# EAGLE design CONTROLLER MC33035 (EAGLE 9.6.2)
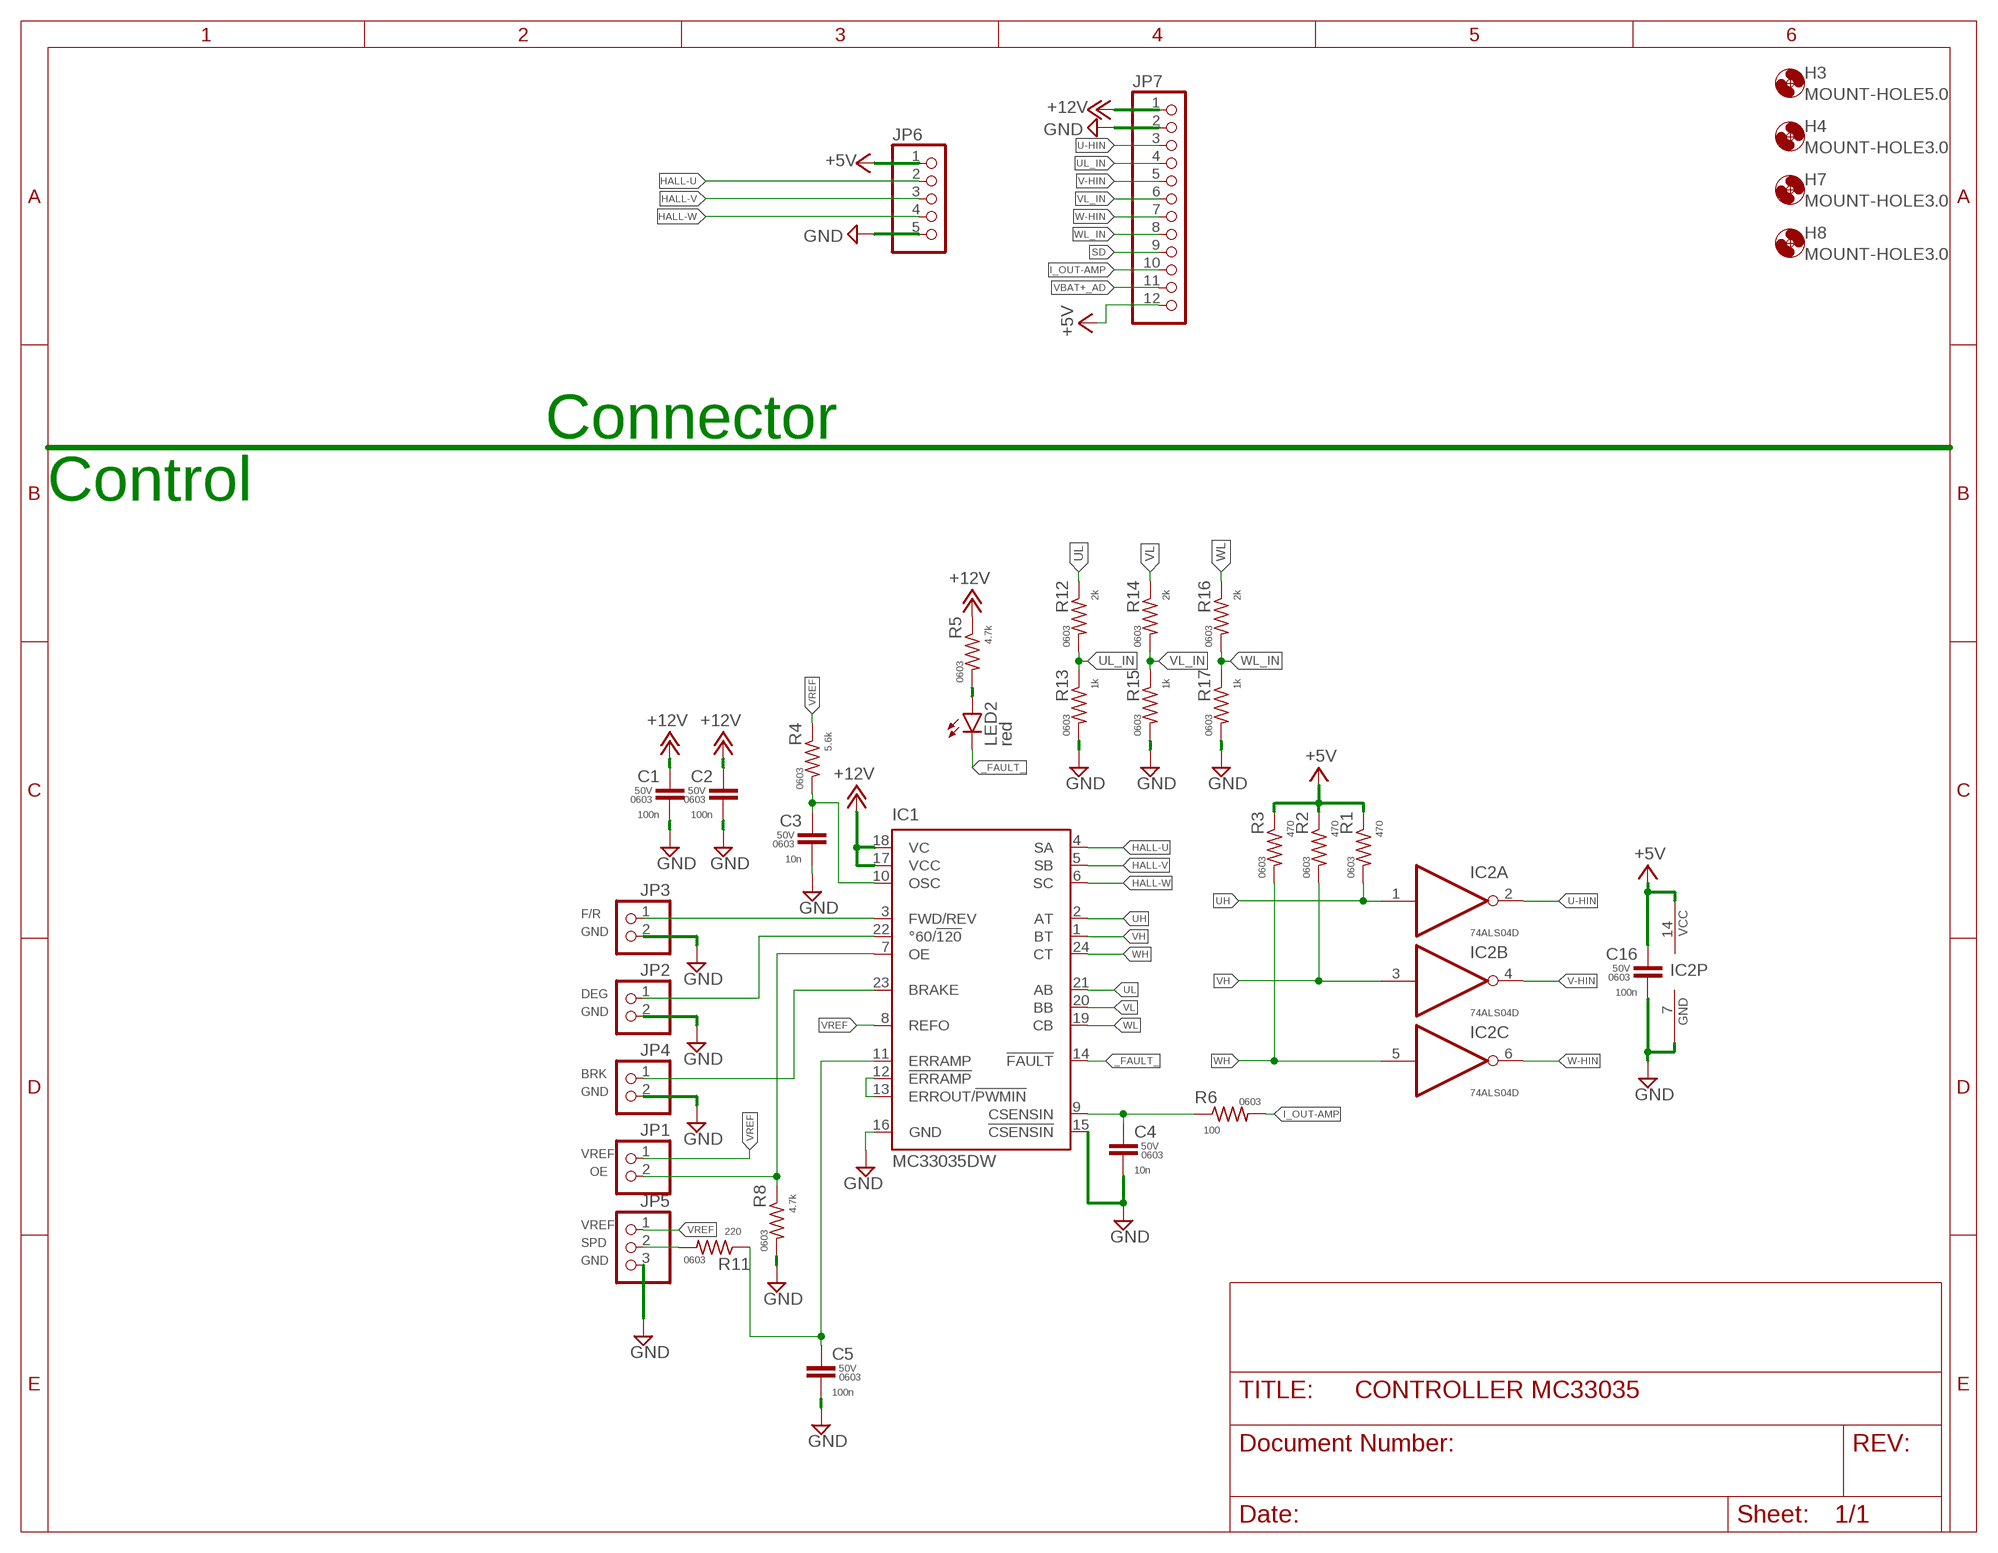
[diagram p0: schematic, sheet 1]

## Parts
C1  100n  C-EUC0603  [C0603]
C2  100n  C-EUC0603  [C0603]
C3  10n  C-EUC0603  [C0603]
C4  10n  C-EUC0603  [C0603]
C5  100n  C-EUC0603  [C0603]
C16  100n  C-EUC0603  [C0603]
H3  MOUNT-HOLE5.0  [5,0]
H4  MOUNT-HOLE3.0  [3,0]
H7  MOUNT-HOLE3.0  [3,0]
H8  MOUNT-HOLE3.0  [3,0]
IC1  MC33035DW  [SO24L]
IC2  74ALS04D  [SO14]
JP1  PINHD-1X2  [1X02]
JP2  PINHD-1X2  [1X02]
JP3  PINHD-1X2  [1X02]
JP4  PINHD-1X2  [1X02]
JP5  PINHD-1X3  [1X03]
JP6  PINHD-1X5  [1X05]
JP7  PINHD-1X12  [1X12]
LED2  red  LEDCHIP-LED0805  [CHIP-LED0805]
R1  470  R-US_R0603  [R0603]
R2  470  R-US_R0603  [R0603]
R3  470  R-US_R0603  [R0603]
R4  5.6k  R-US_R0603  [R0603]
R5  4.7k  R-US_R0603  [R0603]
R6  100  R-US_R0603  [R0603]
R8  4.7k  R-US_R0603  [R0603]
R11  220  R-US_R0603  [R0603]
R12  2k  R-US_R0603  [R0603]
R13  1k  R-US_R0603  [R0603]
R14  2k  R-US_R0603  [R0603]
R15  1k  R-US_R0603  [R0603]
R16  2k  R-US_R0603  [R0603]
R17  1k  R-US_R0603  [R0603]

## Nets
+5V: C16.1 IC2.14(P:VCC) JP6.1 JP7.12 R1.1 R2.1 R3.1
+12V: C1.1 C2.1 IC1.17(VCC) IC1.18(VC) JP7.1 R5.1
_FAULT_: IC1.14(!FAULT) LED2.C
BRK: IC1.23(BRAKE) JP4.1
CSENSE: C4.1 IC1.9(CSENSIN) R6.1
DEG: IC1.22(°60/!120) JP2.1
F/R: IC1.3(FWD/REV) JP3.1
GND: C1.2 C2.2 C3.2 C4.2 C5.2 C16.2 IC1.15(!CSENSIN) IC1.16(GND) IC2.7(P:GND) JP2.2 JP3.2 JP4.2 JP5.3 JP6.5 JP7.2 R8.2 R13.2 R15.2 R17.2
HALL-U: IC1.4(SA) JP6.2
HALL-V: IC1.5(SB) JP6.3
HALL-W: IC1.6(SC) JP6.4
I_OUT-AMP: JP7.10 R6.2
N$2: LED2.A R5.2
N$3: JP5.2 R11.2
N$6: IC1.12(!ERRAMP) IC1.13(ERROUT/!PWMIN)
OE: IC1.7(OE) JP1.2 R8.1
OSC: C3.1 IC1.10(OSC) R4.2
SD: JP7.9
SPD: C5.1 IC1.11(ERRAMP) R11.1
U-HIN: IC2.2(A:O) JP7.3
UH: IC1.2(AT) IC2.1(A:I) R1.2
UL: IC1.21(AB) R12.1
UL_IN: JP7.4 R12.2 R13.1
V-HIN: IC2.4(B:O) JP7.5
VBAT+_AD: JP7.11
VH: IC1.1(BT) IC2.3(B:I) R2.2
VL: IC1.20(BB) R14.1
VL_IN: JP7.6 R14.2 R15.1
VREF: IC1.8(REFO) JP1.1 JP5.1 R4.1
W-HIN: IC2.6(C:O) JP7.7
WH: IC1.24(CT) IC2.5(C:I) R3.2
WL: IC1.19(CB) R16.1
WL_IN: JP7.8 R16.2 R17.1
Unconnected: IC2.8(D:O) IC2.9(D:I) IC2.10(E:O) IC2.11(E:I) IC2.12(F:O) IC2.13(F:I)

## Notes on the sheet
- Connector
- Control

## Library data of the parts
C1-C5 C16 = rcl:C-EU: CAPACITOR, European symbol; SIZE: 0603; SPICEPREFIX: C; VOLTAGE: 50V
H3 H4 H7 H8 = holes:MOUNT-HOLE: MOUNTING HOLE with drill center marker
IC1 = motorola-sensor-driver:*33035: Brushless DC Motor Controller http://onsemi.com; mc33035-d.pdf; MF: ON SEMICONDUCTOR; MPN: MC33035DW; OC_FARNELL: 1652428; OC_NEWARK: 07F4697
IC2 = 74xx-us:74*04: Hex INVERTER
JP1-JP4 = pinhead:PINHD-1X2: PIN HEADER
JP5 = pinhead:PINHD-1X3: PIN HEADER
JP6 = pinhead:PINHD-1X5: PIN HEADER
JP7 = pinhead:PINHD-1X12: PIN HEADER
LED2 = led:LED: LED
R1-R6 R8 R11-R17 = rcl:R-US_: RESISTOR, American symbol; SIZE: 0603; SPICEPREFIX: R

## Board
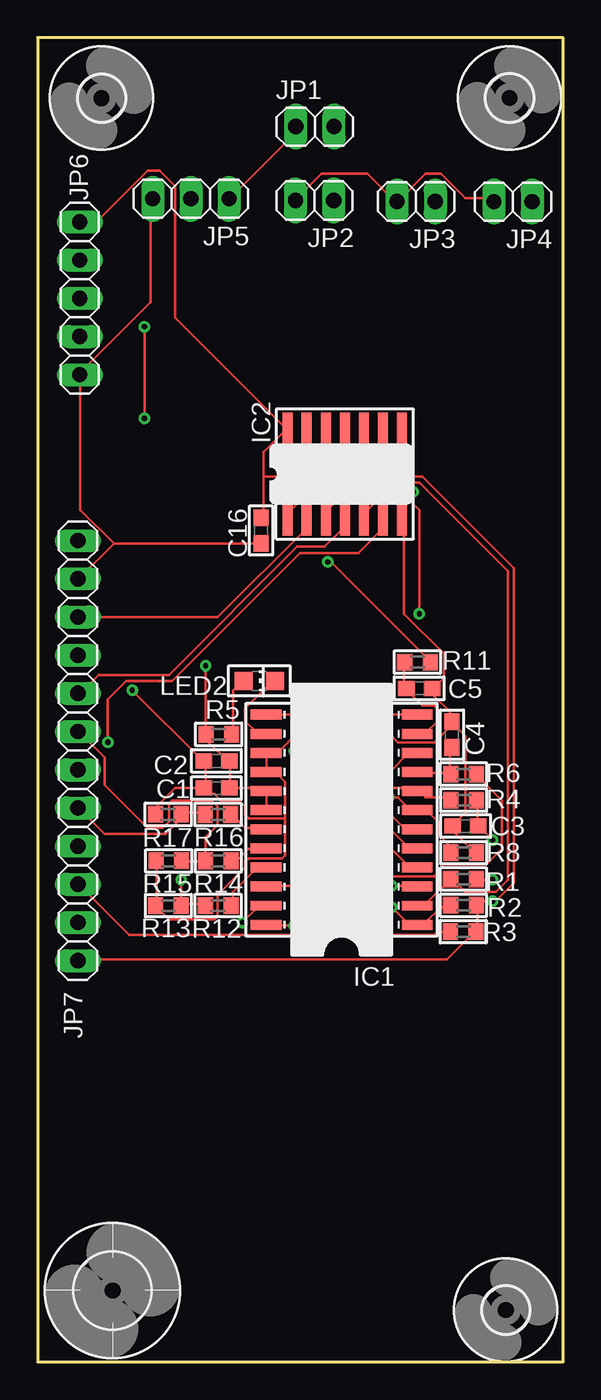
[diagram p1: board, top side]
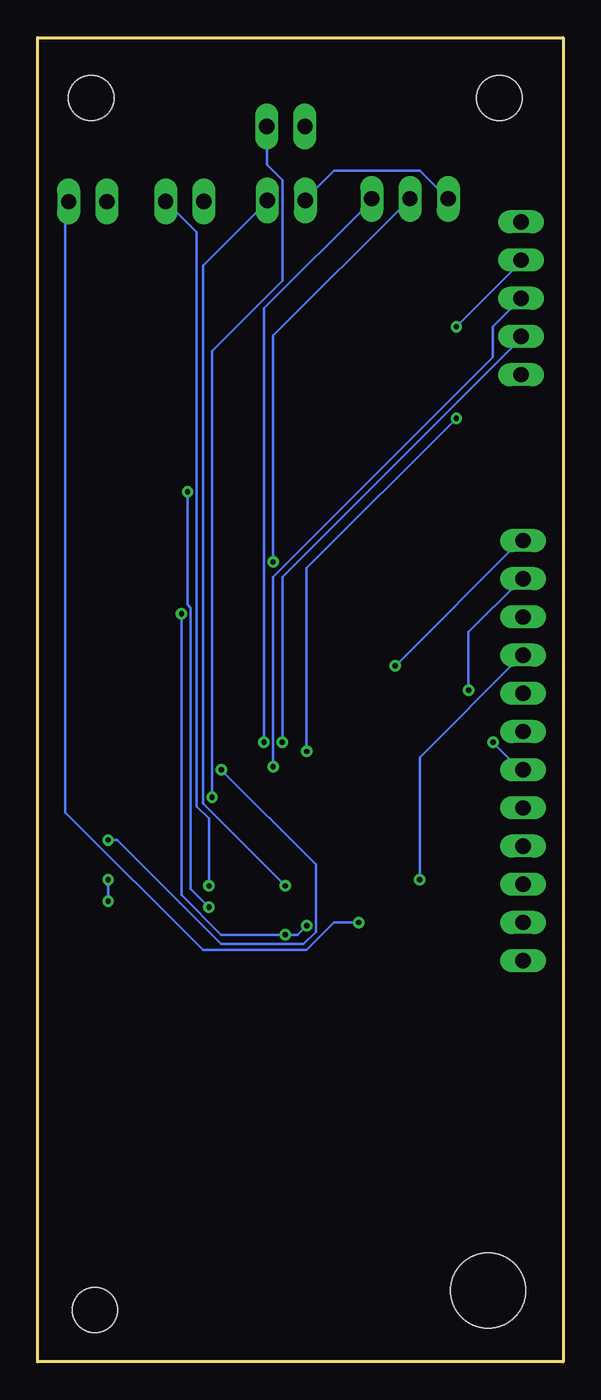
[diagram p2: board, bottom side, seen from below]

Size 34.98 x 88.07 mm. Coordinates in mm from the lower left corner, seen from the top.
Outline: 0,88.07 0,0 34.98,0 34.98,88.07 0,88.07
Copper layers (1*16): Top 0.035mm / dielectric 1.5mm / Bottom 0.035mm
Design rules "default": minimum track width 6mil, minimum drill 0.35mm, track to track 6mil, track to pad 6mil, pad to pad 6mil, via to via 6mil, smd to smd 6mil, copper to edge 40mil, drill to drill 6mil, minimum pad ring 10mil, minimum via ring 8mil, stop-mask expansion 4mil, vias tented up to drill 0mil, thermal gap 10mil

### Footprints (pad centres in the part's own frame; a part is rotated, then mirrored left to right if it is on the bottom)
C0603 = smd 1.1 x 1: 1 -0.85,0; 2 0.85,0
5,0 = hole 5: 0,0
3,0 = hole 3: 0,0
SO24L = smd 0.66 x 2.032: 1 -6.985,-5.029; 2 -5.715,-5.029; 3 -4.445,-5.029; 4 -3.175,-5.029; 5 -1.905,-5.029; 6 -0.635,-5.029; 7 0.635,-5.029; 8 1.905,-5.029; 9 3.175,-5.029; 10 4.445,-5.029; 11 5.715,-5.029; 12 6.985,-5.029; 13 6.985,5.029; 14 5.715,5.029; 15 4.445,5.029; 16 3.175,5.029; 17 1.905,5.029; 18 0.635,5.029; 19 -0.635,5.029; 20 -1.905,5.029; 21 -3.175,5.029; 22 -4.445,5.029; 23 -5.715,5.029; 24 -6.985,5.029
SO14 = smd 0.66 x 2.032: 1 -3.81,-3.073; 2 -2.54,-3.073; 3 -1.27,-3.073; 4 0,-3.073; 5 1.27,-3.073; 6 2.54,-3.073; 7 3.81,-3.073; 8 3.81,3.073; 9 2.54,3.073; 10 1.27,3.073; 11 0,3.073; 12 -1.27,3.073; 13 -2.54,3.073; 14 -3.81,3.073
1X02 = drill 1.016 long: 1 -1.27,0; 2 1.27,0
1X03 = drill 1.016 long: 1 -2.54,0; 2 0,0; 3 2.54,0
1X05 = drill 1.016 long: 1 -5.08,0; 2 -2.54,0; 3 0,0; 4 2.54,0; 5 5.08,0
1X12 = drill 1.016 long: 1 -13.97,0; 2 -11.43,0; 3 -8.89,0; 4 -6.35,0; 5 -3.81,0; 6 -1.27,0; 7 1.27,0; 8 3.81,0; 9 6.35,0; 10 8.89,0; 11 11.43,0; 12 13.97,0
CHIP-LED0805 = smd 1.2 x 1.2: A 0,-1.05; C 0,1.05
R0603 = smd 1 x 1.1: 1 -0.85,0; 2 0.85,0

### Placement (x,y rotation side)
C1  11.9,38.17 180 top
C2  11.9,39.97 180 top
C3  28.48,35.64 180 top
C4  27.58,41.71 90 top
C5  25.39,44.79 0 top
C16  14.87,55.3 270 top
H3  4.99,4.75 0 top
H4  31.15,3.45 0 top
H7  4.25,84.05 0 top
H8  31.41,84.06 0 top
IC1  20.23,36.06 90 top
IC2  20.45,59.04 0 top
JP1  18.45,82.16 0 top
JP2  18.43,77.24 180 top
JP3  25.18,77.18 180 top
JP4  31.64,77.17 180 top
JP5  10.2,77.36 180 top
JP6  2.81,70.74 270 top
JP7  2.68,40.65 270 top
LED2  14.75,45.29 270 top
R1  28.33,32.11 180 top
R2  28.33,30.37 180 top
R3  28.32,28.61 180 top
R4  28.35,37.36 0 top
R5  12.05,41.74 0 top
R6  28.34,39.09 0 top
R8  28.35,33.87 0 top
R11  25.28,46.54 0 top
R12  12.01,30.35 180 top
R13  8.7,30.34 180 top
R14  12.02,33.32 180 top
R15  8.73,33.32 180 top
R16  12,36.41 180 top
R17  8.69,36.41 180 top

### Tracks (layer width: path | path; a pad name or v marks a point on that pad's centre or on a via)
+5V  (via drill 0.35)
  Top 0.152: v30.28,32.07 29.26,32.07 R1.1 | JP7.12 2.84,26.78 27.23,26.78 29.06,28.61 R3.1 29.26,28.82 29.26,30.24 R2.1 29.26,30.44 29.46,30.64 v30.28,30.64 30.48,30.64 31.7,31.86 31.7,52.79 25.6,58.89 15.04,58.89 | 15.04,58.89 15.04,60.52 16.46,61.94 IC2.14 16.46,62.14 9.14,69.46 9.14,78.19 8.13,79.21 7.31,79.21 4.06,75.96 2.84,75.96 JP6.1 | 15.04,58.89 15.04,56.25 C16.1
  Bottom 0.152: v30.28,30.64 v30.28,32.07
+12V  (via drill 0.35)
  Top 0.152: IC1.18 15.24,36.74 15.24,37.96 IC1.17 15.04,38.16 12.8,38.16 C1.1 12.8,38.37 12.8,39.79 C2.1 12.6,39.99 11.38,41.21 11.38,41.62 R5.1 11.18,41.82 v11.18,46.29
  Bottom 0.152: v11.18,46.29 2.84,54.62 JP7.1
_FAULT_
  Top 0.152: LED2.C 15.65,45.28 13.82,43.45 13.82,42.63 14.63,41.82 15.04,41.82 IC1.14
BRK  (via drill 0.35)
  Top 0.152: v13.61,29.22 14.63,30.24 15.04,30.24 IC1.23
  Bottom 0.152: v13.61,29.22 15.24,29.22 17.07,27.39 23.98,27.39 33.12,36.54 33.12,77.1 JP4.1
CSENSE
  Top 0.152: 27.43,39.18 27.43,40.8 C4.1 | 27.43,39.18 25.4,39.18 IC1.9 | 27.43,39.18 R6.1
DEG  (via drill 0.35)
  Top 0.152: v18.49,31.66 15.24,31.66 IC1.22
  Bottom 0.152: v18.49,31.66 23.98,37.15 23.98,72.91 19.71,77.18 JP2.1
F/R  (via drill 0.35)
  Top 0.152: v23.57,31.66 25.2,31.66 IC1.3
  Bottom 0.152: v23.57,31.66 23.57,36.13 24.38,36.94 24.38,75.15 26.42,77.18 JP3.1
GND  (via drill 0.35)
  Top 0.152: R17.2 7.92,36.54 7.92,36.94 9.14,38.16 10.97,38.16 C1.2 | C1.2 11.18,38.37 11.18,39.79 C2.2 10.97,39.99 v6.3,44.67 | R15.2 7.92,33.29 7.92,30.44 R13.2 7.92,30.24 8.74,29.43 11.79,29.43 11.99,29.63 11.99,31.05 13.82,32.88 13.82,33.29 14.02,33.49 16.26,33.49 16.46,33.69 16.46,36.13 | 16.46,36.13 16.46,38.57 15.85,39.18 15.24,39.18 IC1.16 15.24,39.38 15.24,40.4 IC1.15 15.24,40.6 16.05,40.6 17.27,41.82 23.37,41.82 23.98,41.21 26.42,41.21 27.63,42.43 | 16.46,36.13 14.02,36.13 13.82,36.33 13.82,36.94 13.41,37.35 12.19,37.35 11.79,37.76 11.58,37.76 11.18,38.16 C1.2 | R8.2 29.06,33.9 27.43,35.52 C3.2 27.63,35.72 28.45,36.54 28.45,41.62 27.63,42.43 | IC2.7 24.38,55.84 24.38,49.75 27.03,47.1 27.03,45.48 26.42,44.87 C5.2 26.42,44.67 26.42,44.26 27.43,43.24 27.43,42.63 C4.2 27.63,42.43 | JP2.2 17.27,77.38 18.9,79.01 21.95,79.01 23.77,77.18 JP3.2 23.98,77.18 25.81,79.01 26.82,79.01 28.45,77.38 30.28,77.38 JP4.2 | 5.08,54.42 14.83,54.42 C16.2 | 5.08,54.42 2.84,52.18 JP7.2 | 5.08,54.42 2.84,56.65 2.84,65.6 JP6.5 2.84,65.8 7.52,70.47 7.52,77.18 JP5.3
  Bottom 0.152: JP5.3 7.72,77.38 9.55,79.21 15.24,79.21 17.07,77.38 JP2.2 | v6.3,44.67 6.3,48.53 2.84,51.98 JP7.2
HALL-U  (via drill 0.35)
  Top 0.152: v17.07,40.6 24.59,33.08 25.2,33.08 IC1.4 | v7.11,68.85 v7.11,62.75
  Bottom 0.152: v17.07,40.6 17.07,52.79 v7.11,62.75 | v7.11,68.85 2.84,73.11 JP6.2
HALL-V  (via drill 0.35)
  Top 0.152: v19.3,39.59 24.59,34.3 25.2,34.3 IC1.5
  Bottom 0.152: v19.3,39.59 19.3,52.18 4.67,66.81 4.67,68.85 2.84,70.68 JP6.3
HALL-W  (via drill 0.35)
  Top 0.152: v18.69,41.21 24.38,35.52 25.2,35.52 IC1.6
  Bottom 0.152: v18.69,41.21 18.69,52.18 2.84,68.03 JP6.4
I_OUT-AMP
  Top 0.152: R6.2 29.26,38.98 30.89,37.35 30.89,34.1 29.87,33.08 27.03,33.08 26.62,32.68 26.62,32.47 26.42,32.27 21.34,32.27 17.47,28.41 6.1,28.41 2.84,31.66 JP7.10
N$2
  Top 0.152: R5.2 13,41.82 13,44.67 13.61,45.28 LED2.A
N$3  (via drill 0.35)
  Top 0.152: v19.3,53.2 19.51,53.2 26.01,46.7 R11.2
  Bottom 0.152: v19.3,53.2 19.3,68.24 10.36,77.18 JP5.2
N$6
  Top 0.152: IC1.13 15.24,43.04 25.2,43.04 IC1.12
OE  (via drill 0.35)
  Top 0.152: R8.1 27.43,33.9 27.43,34.3 26.62,35.12 26.62,35.93 26.01,36.54 25.4,36.54 IC1.7 25.2,36.74 24.79,36.74 23.98,37.55 v23.37,37.55
  Bottom 0.152: v23.37,37.55 23.37,67.22 18.69,71.89 18.69,78.6 19.71,79.62 19.71,82.05 JP1.2
OSC  (via drill 0.35)
  Top 0.152: R4.2 29.26,37.35 29.26,35.72 C3.1 29.46,35.52 v30.28,34.71 | v22.76,39.38 23.57,39.38 24.59,40.4 25.2,40.4 IC1.10
  Bottom 0.152: v30.28,34.71 29.67,34.71 22.76,27.8 17.27,27.8 16.46,28.61 16.46,33.08 v22.76,39.38
SPD
  Top 0.152: R11.1 24.38,46.49 24.38,44.87 C5.1 24.59,44.67 25.6,43.65 26.42,43.65 26.62,43.45 26.62,42.63 25.81,41.82 25.4,41.82 IC1.11
U-HIN
  Top 0.152: JP7.3 11.99,49.54 17.88,55.44 17.88,55.84 IC2.2
UH
  Top 0.152: IC1.2 25.4,30.44 25.81,30.44 27.43,32.07 R1.2 27.63,32.07 28.45,31.25 30.48,31.25 31.29,32.07 31.29,52.59 25.4,58.48 18.69,58.48 16.66,56.45 16.66,56.04 IC2.1
UL
  Top 0.152: R12.1 13,30.44 13,31.25 14.63,32.88 15.04,32.88 IC1.21
UL_IN  (via drill 0.35)
  Top 0.152: R12.2 10.97,30.44 9.75,30.44 R13.1 9.55,30.44 v9.55,32.07
  Bottom 0.152: v9.55,32.07 9.55,40.2 2.84,46.9 JP7.4
V-HIN
  Top 0.152: IC2.4 20.32,55.84 20.32,55.44 19.1,54.22 17.27,54.22 8.74,45.68 4.06,45.68 2.84,44.46 JP7.5
VH  (via drill 0.35)
  Top 0.152: R2.2 27.43,30.24 26.82,30.24 25.81,29.22 25.4,29.22 IC1.1 25.2,29.22 24.59,29.22 v23.57,30.24 | v24.99,57.87 20.52,57.87 19.3,56.65 19.3,56.04 IC2.3
  Bottom 0.152: v24.99,57.87 24.99,50.36 24.79,50.15 24.79,31.46 v23.57,30.24
VL
  Top 0.152: R14.1 13,33.49 13.41,33.49 14.02,34.1 15.04,34.1 IC1.20
VL_IN
  Top 0.152: R15.1 9.75,33.29 10.97,33.29 R14.2 11.18,33.49 11.18,34.91 11.99,35.72 11.99,36.94 11.58,37.35 8.94,37.35 8.74,37.15 8.74,35.93 8.33,35.52 7.31,35.52 4.47,38.37 4.47,40.2 2.84,41.82 JP7.6
VREF  (via drill 0.35)
  Top 0.152: R4.1 27.43,37.55 25.81,37.55 25.4,37.96 IC1.8 25.2,38.16 22.96,38.16 v19.91,41.21 | JP1.1 17.07,82.05 17.07,81.65 12.8,77.38 JP5.1
  Bottom 0.152: v19.91,41.21 19.91,70.07 12.8,77.18 JP5.1
W-HIN  (via drill 0.35)
  Top 0.152: v4.67,41.21 4.67,44.06 5.89,45.28 8.94,45.28 17.47,53.81 21.34,53.81 22.96,55.44 22.96,55.84 IC2.6
  Bottom 0.152: v4.67,41.21 2.84,39.38 JP7.7
WH  (via drill 0.35)
  Top 0.152: v18.49,28.41 26.42,28.41 26.62,28.61 27.43,28.61 R3.2 | v17.07,29.02 15.24,29.02 IC1.24 | v25.4,49.75 25.4,56.65 24.79,57.26 22.55,57.26 21.74,56.45 21.74,56.04 IC2.5
  Bottom 0.152: v17.07,29.02 17.68,28.41 v18.49,28.41 22.76,28.41 25.4,31.05 v25.4,49.75
WL
  Top 0.152: R16.1 13,36.33 13.82,35.52 15.04,35.52 IC1.19
WL_IN
  Top 0.152: R16.2 10.97,36.54 9.55,36.54 R17.1 9.35,36.33 9.35,35.93 8.53,35.12 4.47,35.12 2.84,36.74 JP7.8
